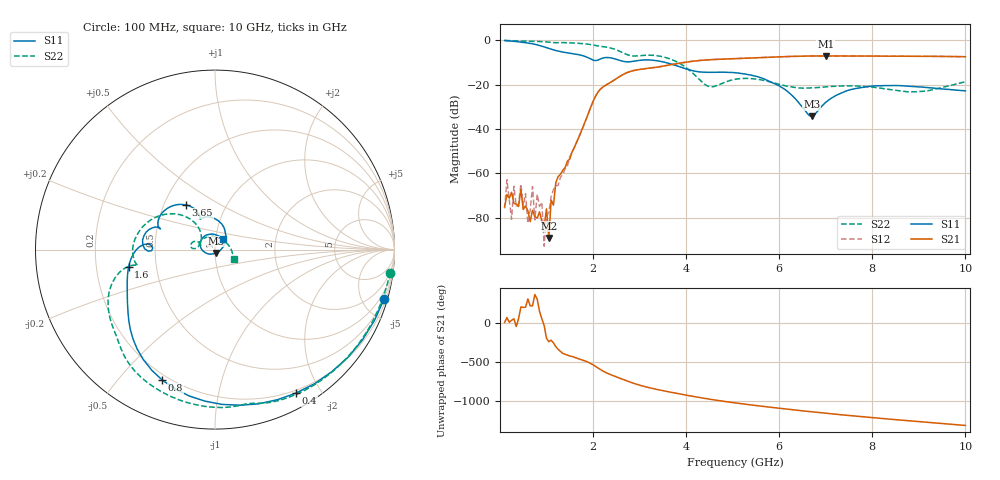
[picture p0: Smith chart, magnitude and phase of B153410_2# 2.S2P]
!  2-Port S-parameters saved by WinCal
! VAR MeasName=S-Parameters (CALIBRATED_DATA) read from VNA (N5245A)
! VAR MeasDate=2016-12-23 9:59:27
! VAR NAME=B153410_2# 2
! VAR FILENAME=B153410_2# 2.S2P
! VAR DATE=2016-12-23 9:59:27
! VAR PHYS_PORTS=1,2
# Hz S DB R 50
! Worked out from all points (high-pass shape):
!   199 points, 100 MHz to 10 GHz, reference 50 ohm
!   highest |S21| = -7.09 dB at 7 GHz (marker M1); lowest = -89.1 dB at 1.05 GHz (marker M2)
!   |S21| within 3 dB of the highest: 3.936 GHz to end of sweep
!   lowest |S11| = -34.2 dB at 6.7 GHz (marker M3), VSWR 1.04, Z = 50.7 - j1.84 ohm
!   |S11| at or under -10 dB: 3.549 GHz to end of sweep
!   |S22| runs from -23.3 to -0.1 dB; largest |S21 - S12| = 0.0024
!   S11 on the Smith chart (normalised r, x): 100 MHz: 0.46, -7.01; 400 MHz: 0.17, -1.70; 800 MHz: 0.18, -0.66; 1.6 GHz: 0.34, -0.09; 3.65 GHz: 0.65, +0.35; 10 GHz: 1.08, +0.13
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1e8  -0.16 -16.2  -75.11 8.8  -75.82 3.4  -0.13 -7.4
1.5e8  -0.25 -23.9  -69.57 70.8  -62.87 16.9  -0.18 -10.9
2.5e8  -0.41 -39.0  -68.53 35.7  -80.69 -148.4  -0.25 -17.6
3e8  -0.52 -46.3  -73.52 54.6  -65.84 18.9  -0.28 -21.0
4e8  -0.74 -60.5  -74.94 57.0  -73.56 12.5  -0.33 -27.6
4.5e8  -0.86 -67.4  -67.15 -153.6  -64.84 127.9  -0.36 -30.9
6e8  -1.28 -87.4  -76.91 -50.1  -82.48 -126.7  -0.45 -40.8
7e8  -1.64 -100.1  -76.61 -138.6  -65.97 -67.2  -0.52 -47.4
7.5e8  -1.87 -106.2  -79.48 5.9  -81.04 153.1  -0.55 -50.7
8e8  -2.12 -112.1  -80.21 -51.2  -69.39 -54.4  -0.59 -53.9
1.05e9  -3.75 -136.6  -89.07 122.1  -77.60 -167.3  -0.87 -70.3
1.2e9  -4.69 -146.6  -64.22 58.3  -65.53 75.2  -1.14 -78.5
1.6e9  -6.17 -168.4  -48.25 -79.0  -48.29 -79.9  -1.30 -103.6
1.75e9  -6.82 -176.9  -40.88 -108.0  -41.04 -108.3  -1.52 -113.5
2.2e9  -8.13 179.3  -21.30 109.5  -21.28 109.6  -2.88 -141.9
3.4e9  -9.35 134.4  -12.09 -133.7  -12.07 -133.9  -7.09 169.2
3.65e9  -10.57 122.8  -11.14 -163.7  -11.14 -163.9  -8.42 152.0
5.05e9  -14.66 100.7  -8.30 57.1  -8.31 57.2  -17.62 175.3
6.7e9  -34.23 -69.4  -7.13 -57.4  -7.14 -57.4  -21.52 166.9
7e9  -27.97 -141.1  -7.09 -75.9  -7.10 -75.8  -21.07 167.0
8.35e9  -20.45 134.0  -7.21 -150.4  -7.20 -150.4  -22.17 111.8
1e10  -22.84 53.1  -7.45 127.8  -7.48 127.9  -18.73 -26.2
